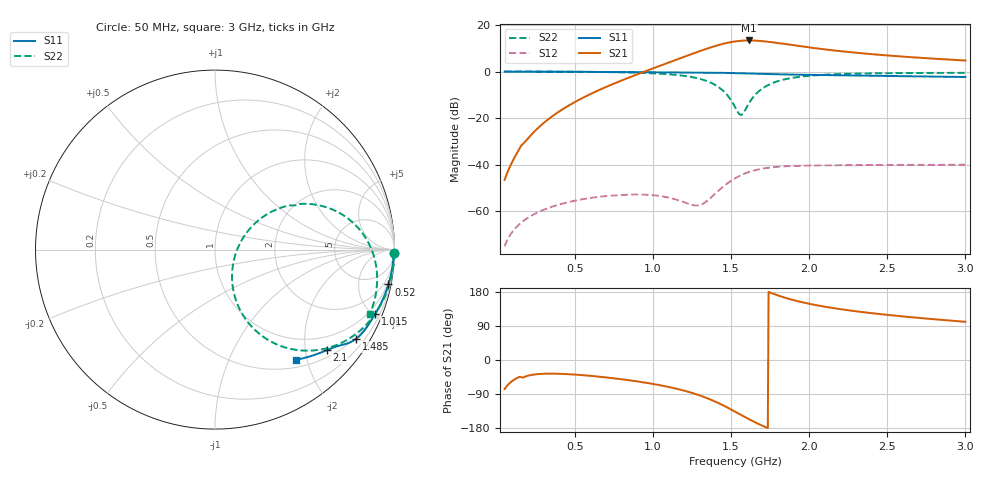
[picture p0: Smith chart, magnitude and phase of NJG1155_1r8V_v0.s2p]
! NJG1155UX2 S-parameter at VDD=1.8V
! Ver.0 2013-06-07
# hz S ma R 50
! freq  magS11  angS11  magS21  angS21  magS12  angS12  magS22  angS22
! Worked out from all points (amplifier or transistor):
!   591 points, 50 MHz to 3 GHz, reference 50 ohm
!   highest |S21| = 13.3 dB at 1.615 GHz (marker M1)
!   |S21| within 3 dB of that: 1.369 GHz to 2.002 GHz (632.9 MHz wide, 37.6 % of centre)
!   unconditionally stable (mu >= 1): 804.9 MHz to end of sweep
!   at 540 MHz: K = 0.50, MSG = 21.7 dB, |S12| = -55.0 dB
!   at 1.525 GHz: K = 3.23, MAG = 21.4 dB, |S12| = -45.9 dB
!   at 3 GHz: K = 1.78, MAG = 17.3 dB, |S12| = -40.1 dB
!   lowest NFmin = 0.43 dB at 745 MHz
!   S11 on the Smith chart (normalised r, x): 50 MHz: open; 520 MHz: 1, -10; 1.015 GHz: 0.54, -5.15; 1.485 GHz: 0.46, -3.39; 2.1 GHz: 0.65, -2.45; 3 GHz: 0.62, -1.81
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5e7  0.9956 -1.1  0.004685 -76.7  0.0001765 89.7  0.9999 -1.2
1.5e8  0.9948 -3.3  0.02359 -44.6  0.0005414 87.8  0.999 -3.6
2.25e8  0.9936 -4.9  0.04525 -39.2  0.0008097 85.9  0.9979 -5.5
5.2e8  0.9855 -11.4  0.2401 -39.1  0.001728 79.1  0.9871 -13.2
5.45e8  0.9845 -11.9  0.2657 -39.9  0.001792 78.5  0.9855 -13.9
8.1e8  0.9729 -17.5  0.6635 -51.4  0.002233 72.2  0.9585 -22.6
1.015e9  0.9621 -21.8  1.219 -64.3  0.002169 69.8  0.91 -31.7
1.035e9  0.9611 -22.2  1.292 -65.8  0.00213 69.9  0.9026 -32.8
1.18e9  0.9538 -25.2  1.958 -78.8  0.001635 77.9  0.8227 -42.2
1.29e9  0.9483 -27.6  2.67 -92.2  0.001328 111.4  0.7086 -51.8
1.405e9  0.9401 -30.3  3.587 -111.0  0.002491 148.4  0.4978 -63.6
1.485e9  0.9302 -32.3  4.196 -127.3  0.004143 148.7  0.2844 -67.2
1.525e9  0.9234 -33.3  4.427 -136.1  0.00506 144.9  0.1734 -56.9
1.565e9  0.9155 -34.2  4.58 -145.2  0.005952 139.9  0.1169 -13.2
1.615e9  0.905 -35.2  4.647 -156.3  0.006946 132.7  0.2095 29.3
1.695e9  0.8884 -36.6  4.512 -172.5  0.008126 121.4  0.4189 32.9
1.805e9  0.87 -38.1  4.077 169.7  0.009001 108.7  0.6282 23.2
1.9e9  0.8577 -39.4  3.671 158.0  0.009345 100.6  0.7381 15.2
2.02e9  0.8448 -41.0  3.23 146.7  0.009545 93.3  0.8197 7.2
2.1e9  0.8371 -42.1  2.989 140.6  0.009619 89.7  0.8533 2.9
2.51e9  0.801 -47.6  2.2 118.7  0.009817 79.1  0.922 -11.7
3e9  0.7625 -53.6  1.724 100.8  0.009941 74.4  0.9346 -22.6
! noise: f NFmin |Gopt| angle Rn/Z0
5e+07  1.387  0.9746  1.474  12.65
3.75e+08  0.5166  0.921  8.145  1.391
7.05e+08  0.4275  0.8847  14.25  0.7921
1.03e+09  0.4396  0.8613  20.09  0.6441
1.36e+09  0.4796  0.8351  25.52  0.5657
1.685e+09  0.5325  0.8118  31.19  0.5331
2.015e+09  0.5967  0.7885  36.94  0.5107
2.34e+09  0.669  0.7658  42.57  0.4935
2.67e+09  0.752  0.7434  48.22  0.479
3e+09  0.8463  0.7214  53.76  0.4667
